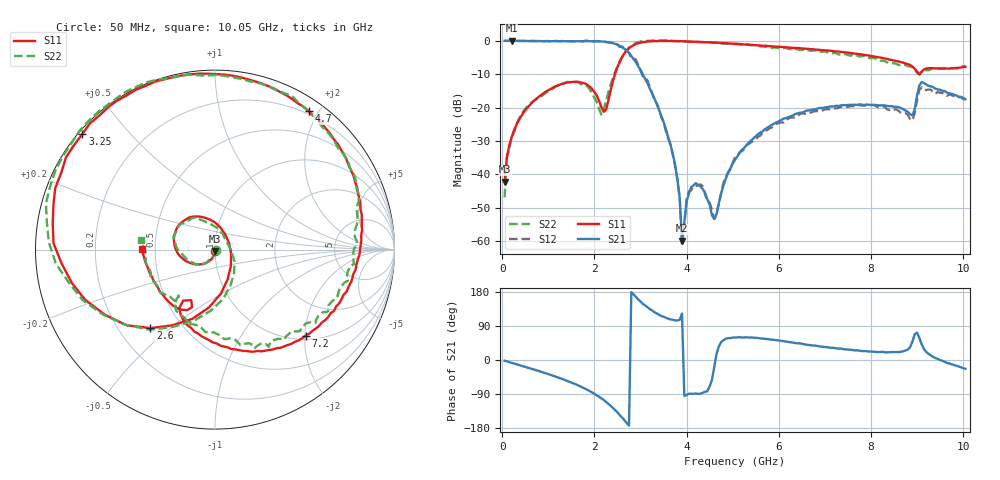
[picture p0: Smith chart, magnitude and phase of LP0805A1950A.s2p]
! AVX THIN FILM OPERATION
! 0805 Size Low Pass Filter P/N  LP0805A1950AWTR
! Network Analyzer HP8720ES.07.64: Feb 23, 2000 Serial No. US39172382
! Hewlett-Packard
!  2 Feb 2003  04:20:02
! Frequency  S11  S21  S12  S22
# HZ  S  DB R  50
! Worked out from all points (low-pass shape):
!   201 points, 50 MHz to 10.05 GHz, reference 50 ohm
!   highest |S21| = -0.01 dB at 200 MHz (marker M1); lowest = -59.8 dB at 3.9 GHz (marker M2)
!   |S21| within 3 dB of the highest: start of sweep to 2.695 GHz
!   lowest |S11| = -42.2 dB at 50 MHz (marker M3), VSWR 1.02, Z = 50.1 - j0.773 ohm
!   |S11| at or under -10 dB: start of sweep to 2.446 GHz; 9.039165 GHz to 9.057637 GHz (18.47 MHz wide, 0.204 % of centre)
!   |S22| runs from -46.9 to 0.1 dB; largest |S21 - S12| = 0.066
!   S11 on the Smith chart (normalised r, x): 50 MHz: 1.00, -0.02; 2.6 GHz: 0.33, -0.43; 3.25 GHz: 0.01, +0.37; 4.7 GHz: 0.16, +1.87; 7.2 GHz: 1.09, -2.02; 10.05 GHz: 0.42, +0.00
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5e7  -42.16 -81.6  -0.02 -1.9  -0.02 -1.9  -46.87 -7.0
1e8  -34.95 -92.6  -0.03 -3.6  -0.01 -3.7  -34.45 -92.5
2e8  -28.94 -101.3  -0.01 -7.3  -0.04 -7.4  -29.15 -102.9
6.5e8  -18.44 -136.2  -0.09 -23.7  -0.05 -23.7  -18.30 -135.3
1.75e9  -12.62 134.2  -0.15 -72.8  -0.25 -73.0  -13.20 132.6
2.15e9  -19.84 56.2  -0.24 -101.1  -0.22 -101.6  -22.10 30.9
2.6e9  -4.94 -129.4  -1.91 -151.7  -1.75 -149.7  -4.80 -129.0
2.9e9  -0.91 177.8  -6.41 166.5  -5.66 165.1  -0.66 177.4
3.25e9  -0.17 138.9  -15.67 131.0  -15.68 124.6  0.04 138.7
3.4e9  -0.07 126.8  -20.60 119.5  -20.41 115.2  0.04 126.0
3.75e9  -0.10 103.8  -37.12 104.6  -37.42 105.1  -0.12 102.5
3.85e9  -0.12 98.0  -47.07 106.0  -47.10 105.8  -0.19 96.1
3.9e9  -0.14 95.2  -59.78 122.6  -61.44 136.7  -0.26 93.2
4.05e9  -0.21 87.0  -45.67 -89.1  -44.97 -98.2  -0.30 84.6
4.7e9  -0.62 55.9  -48.61 35.8  -48.67 34.0  -0.66 53.0
5.05e9  -0.89 40.6  -35.59 59.2  -34.87 56.2  -1.00 36.6
6.75e9  -2.55 -27.2  -20.57 38.2  -21.20 38.4  -2.88 -28.5
7.2e9  -3.15 -43.5  -19.64 31.8  -20.24 30.9  -3.66 -43.8
8.4e9  -5.64 -89.1  -19.59 20.6  -20.74 17.2  -6.71 -90.8
8.9e9  -7.72 -117.6  -22.36 48.4  -23.82 43.3  -7.86 -122.2
9.1e9  -9.24 -111.8  -12.35 41.8  -13.91 35.1  -9.35 -126.9
1.005e10  -7.79 179.8  -17.50 -23.2  -17.45 -20.3  -7.58 172.3
